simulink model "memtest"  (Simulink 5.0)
settings: Solver=ode45  StartTime=0.0  StopTime=270  RelTol=1e-3
undefined symbols (not defined in the file or in its folder): Bit, Location, Lower, tmp3, Width
libraries: xbsIndex_r3 x20, ADlibrary x3

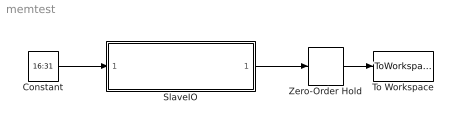
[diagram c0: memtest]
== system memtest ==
  Constant : Constant  Value=16:31
  SlaveIO : Subsystem
  To Workspace : ToWorkspace  VariableName=simout  SampleTime=-1  SaveFormat=Structure
  Zero-Order Hold : ZeroOrderHold  SampleTime=36
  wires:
  Constant/1 -> SlaveIO/1(Vector Input)
  SlaveIO/1(Vector Output) -> Zero-Order Hold/1
  Zero-Order Hold/1 -> To Workspace/1

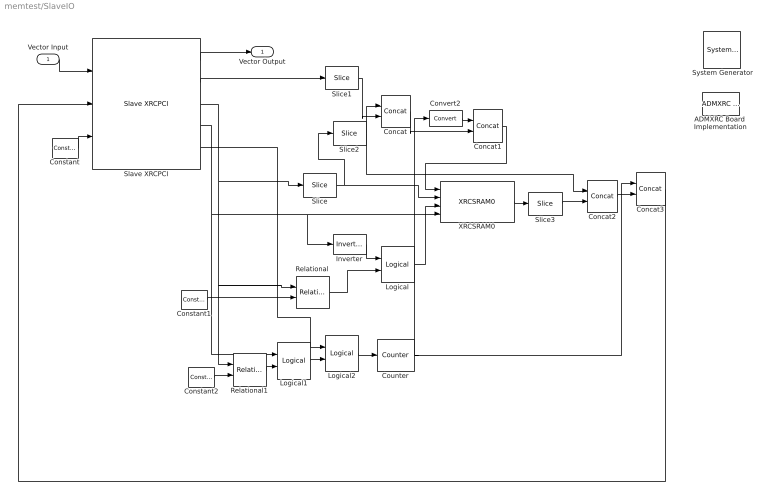
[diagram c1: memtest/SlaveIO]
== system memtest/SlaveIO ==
  Vector Input : Inport
  " System Generator" : xbsIndex_r3/ System Generator  Tag=genX  xilinxfamily=Virtex2  part=xc2v6000  speed=-4  package=ff1152  synthesis_tool=XST  directory=e:/tmp3  testbench=off  simulink_period=1  sysclk_period=10  incr_netlist=off  trim_vbits=According to Block Masks  dbl_ovrd=According to Block Masks  core_generation=According to Block Masks  run_coregen=off  deprecated_control=off  eval_field=0
  ADMXRC Board  Implementation : ADlibrary/Miscellaneous/ADMXRC Board  Implementation  board=XRCII  run_synth=on  make_clean=off  lvds_io_std=3.3v  clock_source=MCLK
  Concat{,1..3} (4 alike) : xbsIndex_r3/Concat  num_inputs=2  explicit_period=off  period=1  dbl_ovrd=off
  Constant : xbsIndex_r3/Constant  const=1  arith_type=Unsigned  n_bits=1  bin_pt=0  explicit_period=on  period=1  dbl_ovrd=off
  Constant1 : xbsIndex_r3/Constant  const=32768  arith_type=Unsigned  n_bits=22  bin_pt=0  explicit_period=on  period=1  dbl_ovrd=off
  Constant2 : xbsIndex_r3/Constant  const=0  arith_type=Unsigned  n_bits=22  bin_pt=0  explicit_period=on  period=1  dbl_ovrd=off
  Convert2 : xbsIndex_r3/Convert  arith_type=Unsigned  n_bits=20  bin_pt=0  quantization=Truncate  overflow=Wrap  latency=0  explicit_period=on  period=1  dbl_ovrd=off  inserted_by_tool=off
  Counter : xbsIndex_r3/Counter  cnt_type=Free Running  n_bits=8  bin_pt=0  arith_type=Unsigned  start_count=0  cnt_to=Inf  cnt_by_val=1  operation=Up  explicit_period=off  period=1  load_pin=off  rst=on  en=off  dbl_ovrd=off  use_rpm=off  gen_core=on
  Inverter : xbsIndex_r3/Inverter  latency=0  explicit_period=off  period=1  en=off  dbl_ovrd=off
  Logical : xbsIndex_r3/Logical  logical_function=AND  inputs=2  precision=Full  arith_type=Unsigned  n_bits=8  bin_pt=2  align_bp=on  latency=0  explicit_period=off  period=1  en=off  dbl_ovrd=off
  Logical1 : xbsIndex_r3/Logical  logical_function=AND  inputs=2  precision=Full  arith_type=Unsigned  n_bits=8  bin_pt=2  align_bp=on  latency=0  explicit_period=off  period=1  en=off  dbl_ovrd=off
  Logical2 : xbsIndex_r3/Logical  logical_function=OR  inputs=2  precision=Full  arith_type=Unsigned  n_bits=8  bin_pt=2  align_bp=on  latency=0  explicit_period=off  period=1  en=off  dbl_ovrd=off
  Relational : xbsIndex_r3/Relational  mode=a<b  latency=0  explicit_period=off  period=1  en=off  dbl_ovrd=off
  Relational1 : xbsIndex_r3/Relational  mode=a=b  latency=0  explicit_period=off  period=1  en=off  dbl_ovrd=off
  Slave XRCPCI : ADlibrary/PCI/Slave XRCPCI  no_inputs=16  no_outputs=16  circuit_lag=1  decode_delay=0
  Slice : xbsIndex_r3/Slice  mode=Lower Bit Location + Width  nbits=20  bit1=0  base1=MSB of Input  bit0=0  base0=LSB of Input  boolean_output=off  explicit_period=off  period=1  dbl_ovrd=off
  Slice1 : xbsIndex_r3/Slice  mode=Lower Bit Location + Width  nbits=8  bit1=0  base1=MSB of Input  bit0=0  base0=LSB of Input  boolean_output=off  explicit_period=off  period=1  dbl_ovrd=off
  Slice2 : xbsIndex_r3/Slice  mode=Lower Bit Location + Width  nbits=4  bit1=0  base1=MSB of Input  bit0=0  base0=LSB of Input  boolean_output=off  explicit_period=off  period=1  dbl_ovrd=off
  Slice3 : xbsIndex_r3/Slice  mode=Lower Bit Location + Width  nbits=20  bit1=0  base1=MSB of Input  bit0=0  base0=LSB of Input  boolean_output=off  explicit_period=off  period=1  dbl_ovrd=off
  XRCSRAM0 : ADlibrary/Memory/XRCSRAM0
  Vector Output : Outport
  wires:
  Slave XRCPCI/1 -> Vector Output/1
  Vector Input/1 -> Slave XRCPCI/1
  Slave XRCPCI/3 -> Slice/1, Relational/1, Relational1/1
  Constant/1 -> Slave XRCPCI/3
  Slice/1 -> Slice2/1, XRCSRAM0/2
  Slave XRCPCI/4 -> Inverter/1, XRCSRAM0/4, Logical1/1
  Constant1/1 -> Relational/2
  Inverter/1 -> Logical/1
  Logical/1 -> XRCSRAM0/3
  Slave XRCPCI/2 -> Slice1/1
  Slice2/1 -> Concat2/1, Concat/1
  Concat/1 -> Concat1/2
  Concat1/1 -> XRCSRAM0/1
  XRCSRAM0/1 -> Slice3/1
  Slice3/1 -> Concat2/2
  Concat2/1 -> Concat3/2
  Slice1/1 -> Concat/2
  Constant2/1 -> Relational1/2
  Convert2/1 -> Concat1/1
  Counter/1 -> Convert2/1, Concat3/1
  Relational1/1 -> Logical1/2
  Relational/1 -> Logical/2
  Logical1/1 -> Logical2/2
  Logical2/1 -> Counter/1
  Slave XRCPCI/5 -> Logical2/1
  Concat3/1 -> Slave XRCPCI/2
